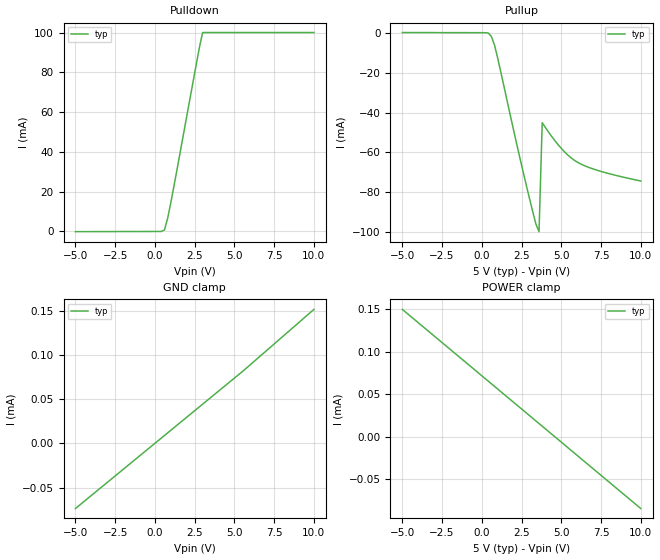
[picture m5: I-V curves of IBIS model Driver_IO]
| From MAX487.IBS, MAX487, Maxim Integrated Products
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|   Driver Input/Output A & B
[Model]   Driver_IO
|Signals   A, B
Model_type   I/O
Vinl = 0.8V
Vinh = 2.0V
C_comp   0.538pF   NA   NA
[Temperature Range]   25   -40   85
[Voltage Range]   5.00V   4.75V   5.25V
[Pullup Reference]   5.00V   4.75V   5.25V
[Pulldown Reference]   0.00V   0.00V   0.00V
[POWER Clamp Reference]   5.00V   4.75V   5.25V
[GND Clamp Reference]   0.00V   0.00V   0.00V
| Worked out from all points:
|   slope of the pulldown table from 0 to 0.75 V, typ, clamps not added: 145 ohm
|   slope of the pullup table from 0 to 0.75 V, typ, clamps not added: 147 ohm
[Pullup]
| Note that the[Pullup]voltage table is referenced to Vcc
| and is calculated using Vtable=Vcc - Vmeasured.
| V(V)  I(typ)   I(min)  I(max)
-5V       149.9uA    NA         NA
200mV     68.32uA    NA         NA
600mV     -1.764mA   NA         NA
1V        -12.72mA   NA         NA
3V        -83.12mA   NA         NA
3.4V      -95.86mA   NA         NA
3.6V      -99.73mA   NA         NA
3.8V      -45.08mA   NA         NA
5V        -57.96mA   NA         NA
6V        -64.83mA   NA         NA
7.4V      -69.28mA   NA         NA
10V       -74.33mA   NA         NA
[Pulldown]
| Note that the[Pulldown]voltage table is referenced to Gnd.
| Also, the Semiconductor Parameter Analyzer (Force and Sense)
| clamps the supply current to 100mA to protect the system.
| V(V)  I(typ)   I(min)  I(max)
-5V       -84.96uA   NA         NA
400mV     949.6nA    NA         NA
600mV     776.2uA    NA         NA
800mV     6.629mA    NA         NA
1V        14.52mA    NA         NA
2.8V      92.55mA    NA         NA
3V        100mA      NA         NA
10V       100mA      NA         NA
[POWER_clamp]
| Note that the[POWER_clamp]voltage table is referenced to Vcc
| and is calculated using Vtable=Vcc - Vmeasured.
| V(V)  I(typ)   I(min)  I(max)
-5V       149.9uA    NA         NA
-4V       134.3uA    NA         NA
-3.2V     121.8uA    NA         NA
10V       -84.96uA   NA         NA
[GND_clamp]
| Note that the[GND_clamp]voltage table is referenced to Gnd.
| V(V)  I(typ)   I(min)  I(max)
-5V       -73.75uA   NA         NA
5.4V      79.65uA    NA         NA
6.2V      92.01uA    NA         NA
10V       151.4uA    NA         NA
[Ramp]
| variable   typ   min   max
dV/dt_r   2.81/0.93uS   NA   NA
dV/dt_f   2.58/0.58uS   NA   NA
R_load = 5Kohms
|End [Model] Driver_IO
|End [Component] MAX487
